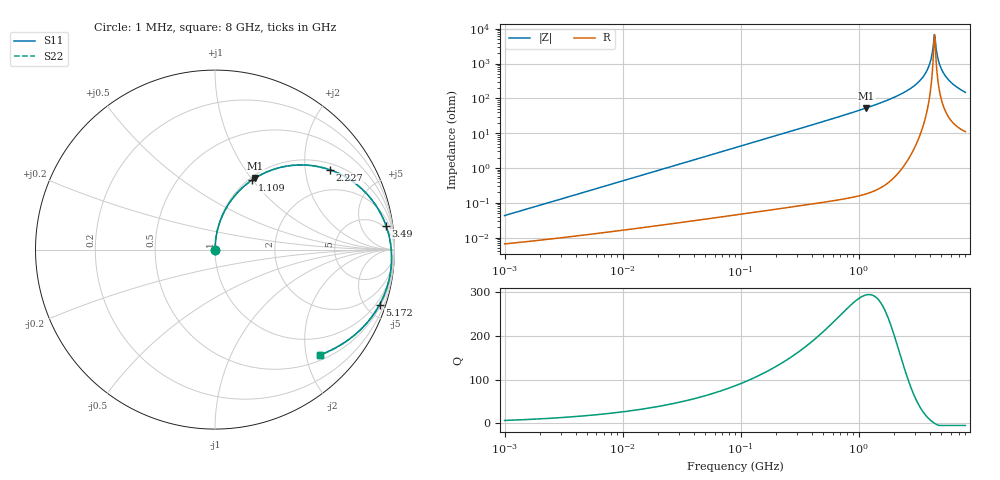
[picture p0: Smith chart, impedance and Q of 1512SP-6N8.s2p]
# MHz  S  MA  R  50
!Freq  MagS11  AngS11  MagS21  AngS21  MagS12  AngS12  MagS22  AngS22
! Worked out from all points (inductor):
!   801 points, 1 MHz to 8 GHz, reference 50 ohm
!   read as one part in series: L = 6.79 nH near 1.046 MHz
!   highest Q = 294 at 1.16 GHz (marker M1), where L = 7.31 nH
!   self-resonance near 4.37 GHz
!   S11 on the Smith chart (normalised r, x): 1 MHz: 1.00, +0.00; 1.109 GHz: 1.04, +1.00; 2.227 GHz: 1.20, +2.71; 3.49 GHz: 4, +13; 5.172 GHz: 0.65, -6.09; 8 GHz: 0.61, -2.28
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1  0.000418 80.9  0.9999 -0.0  0.9999 -0.0  0.000418 80.9
4.507347  0.001864 86.3  0.9999 -0.1  0.9999 -0.1  0.001864 86.3
20.08917  0.008293 88.0  0.9997 -0.5  0.9997 -0.5  0.008293 88.0
89.53707  0.03694 87.0  0.9989 -2.3  0.9989 -2.3  0.03693 87.0
403.5746  0.1656 79.5  0.9853 -10.2  0.9853 -10.2  0.1656 79.5
715.8207  0.2905 71.7  0.9557 -18.0  0.9557 -18.0  0.2904 71.7
1109.493  0.4399 61.9  0.8965 -27.9  0.8965 -27.9  0.4398 61.9
1160.498  0.4584 60.6  0.8872 -29.2  0.8872 -29.2  0.4583 60.6
1798.725  0.6673 45.0  0.742 -44.8  0.742 -44.8  0.6671 45.0
2226.819  0.7791 34.8  0.622 -54.8  0.622 -54.8  0.779 34.8
2883.534  0.9007 20.2  0.4214 -69.0  0.4214 -69.0  0.9006 20.2
3490.481  0.9623 8.0  0.238 -79.8  0.238 -79.8  0.9622 8.0
3905.578  0.9813 0.5  0.1218 -84.2  0.1218 -84.2  0.9813 0.5
4039.479  0.9843 -1.8  0.08662 -83.8  0.08662 -83.8  0.9842 -1.8
4225.182  0.9861 -4.9  0.04065 -76.0  0.04065 -76.0  0.9861 -4.9
4370.04  0.986 -7.2  0.01433 -19.9  0.01433 -19.9  0.986 -7.2
4519.865  0.9846 -9.4  0.03521 55.6  0.03521 55.6  0.9846 -9.4
4727.651  0.9807 -12.5  0.0797 65.9  0.0797 65.9  0.9809 -12.5
4835.1  0.978 -14.0  0.1022 66.6  0.1022 66.6  0.9782 -14.0
5172.321  0.9669 -18.5  0.1684 65.1  0.1684 65.1  0.9672 -18.5
6191.069  0.9195 -30.0  0.3289 55.7  0.3289 55.7  0.92 -30.0
8000  0.8289 -45.0  0.504 41.0  0.504 41.0  0.8302 -45.0
